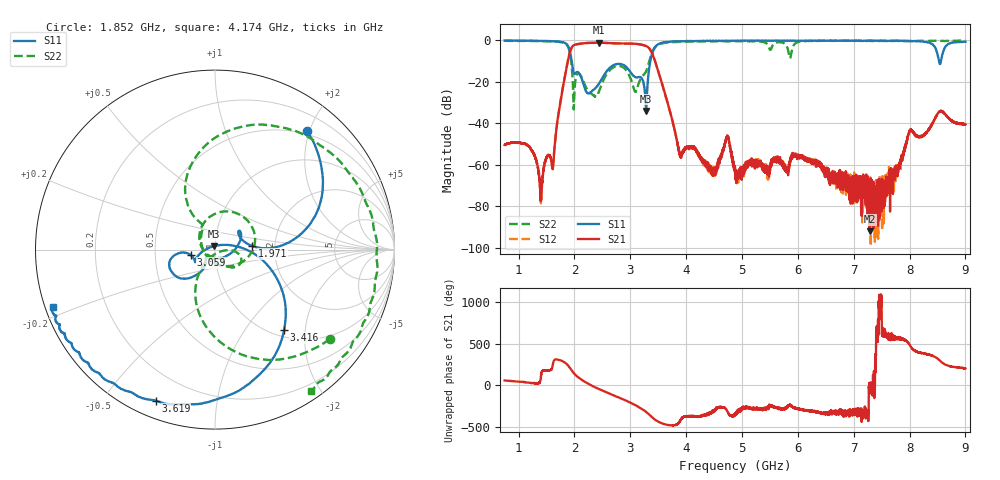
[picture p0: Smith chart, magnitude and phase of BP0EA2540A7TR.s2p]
!Agilent Technologies,E8358A,US41080443,A.07.50.56
!Agilent E8358A: A.07.50.56
!Date: Friday, November 20, 2015 10:53:29
!Correction: S11(Full 2 Port(1,2))
!S21(Full 2 Port(1,2))
!S12(Full 2 Port(1,2))
!S22(Full 2 Port(1,2))
!S2P File: Measurements: S11, S21, S12, S22:
# Hz S  dB  R 50
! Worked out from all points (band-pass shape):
!   6401 points, 750 MHz to 9 GHz, reference 50 ohm
!   highest |S21| = -1.08 dB at 2.435 GHz (marker M1); lowest = -92.0 dB at 7.287 GHz (marker M2)
!   |S21| within 3 dB of the highest: 1.938 GHz to 3.347 GHz (1.408 GHz wide, 53.3 % of centre)
!   lowest |S11| = -34.0 dB at 3.283 GHz (marker M3), VSWR 1.04, Z = 49.2 + j1.83 ohm
!   |S11| at or under -10 dB: 1.951 GHz to 3.359 GHz (1.408 GHz wide, 53 % of centre); 8.526899 GHz to 8.56244 GHz (35.54 MHz wide, 0.416 % of centre)
!   |S22| runs from -33.3 to -0.1 dB; largest |S21 - S12| = 0.0057
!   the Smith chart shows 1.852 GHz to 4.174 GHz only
!   S11 on the Smith chart (normalised r, x): 1.852 GHz: 0.44, +1.95; 1.971 GHz: 1.52, +0.06; 3.059 GHz: 0.76, -0.05; 3.416 GHz: 1.13, -1.55; 3.619 GHz: 0.07, -0.68; 4.174 GHz: 0.02, -0.17
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7.5e8  -0.05 159.7  -50.36 55.9  -50.35 56.2  -0.16 132.8
1.407422e9  -0.22 127.9  -74.49 139.8  -74.05 137.6  -0.32 71.6
1.620117e9  -0.38 107.2  -60.24 -89.5  -60.05 -91.0  -0.49 37.4
1.852148e9  -1.55 52.4  -13.99 -101.0  -14.04 -101.1  -1.82 -38.0
1.970742e9  -13.62 5.5  -2.66 158.4  -2.70 158.5  -20.23 -126.8
2.12543e9  -18.10 7.5  -1.46 65.4  -1.50 65.4  -17.49 -48.0
2.434805e9  -21.03 -126.4  -1.08 -46.8  -1.12 -46.8  -24.99 -162.4
2.804766e9  -11.30 -157.3  -1.48 -152.2  -1.51 -152.3  -12.33 33.6
3.058711e9  -17.16 -167.4  -1.55 130.7  -1.59 130.6  -22.90 -95.3
3.283008e9  -33.99 111.8  -2.67 38.3  -2.71 38.3  -14.92 119.6
3.415781e9  -4.58 -49.3  -7.86 -41.3  -7.85 -41.2  -4.31 91.9
3.500859e9  -1.80 -83.9  -14.77 -80.4  -14.87 -80.0  -2.04 57.9
3.619453e9  -0.87 -111.4  -25.54 -111.7  -25.51 -111.3  -1.17 24.2
3.890156e9  -0.43 -142.4  -55.18 -74.1  -55.29 -74.2  -0.66 -22.2
4.17375e9  -0.35 -160.5  -52.51 -21.9  -53.32 -18.7  -0.45 -55.9
4.738359e9  -0.19 176.8  -45.99 45.4  -46.53 43.9  -0.50 -102.1
4.875e9  -0.15 172.2  -61.93 6.1  -62.58 6.5  -0.34 -110.8
6.25043e9  -0.07 165.5  -58.55 48.3  -57.77 42.5  -0.28 -170.8
7.286836e9  -0.10 138.4  -92.01 5.8  -73.06 0.7  -0.24 162.1
7.625859e9  -0.17 125.1  -68.12 -151.0  -64.58 -150.0  -0.31 154.5
8.019023e9  -0.26 111.2  -43.19 105.8  -43.02 105.5  -0.34 143.9
9e9  -0.66 93.9  -40.44 -158.6  -40.59 -157.7  -0.13 118.9
